TYPE "ST_SystemDataRef"
VERSION : 0.1


  STRUCT
   abyInputData : ARRAY  [1 .. 104 ] OF //This array contains the mapped raw input data
   BYTE ;
   abyOutputData : ARRAY  [1 .. 104 ] OF //This array contains the mapped raw output data
   BYTE ;
   stConnectionSettings : "ST_ConnectionSettings";	//This structure contains all data required for the connection
   xConnected : BOOL ;	//Connection established | FALSE: No connection established | TRUE: Connection es
   xStatusOfConnection : BOOL ;	//Status of the communication module | FALSE: No connection established | TRUE: C
   byActualComMode : BYTE ;	//Actual communication mode | 0x00 = Acyclic communication mode | 0x01 = Cyclic c
   byActualAccessType : BYTE ;	//Actual access type | 0x00 = Read object | 0x01 = Write object
   stAcyclicReadRequest : "ST_AcyclicReadRequest";	//This structure contains all data required to create a acyclic read request
   stAcyclicReadResponse : "ST_AcyclicReadResponse";	//This structure contains all data required to parse a acyclic read response
   stAcyclicWriteRequest : "ST_AcyclicWriteRequest";	//This structure contains all data required to create a acyclic write request
   stAcyclicWriteResponse : "ST_AcyclicWriteResponse";	//This structure contains all data required to parse a acyclic write response
   stCyclicRequest : "ST_CyclicRequest";	//This structure contains all data required to create a cyclic request
   stCyclicResponse : "ST_CyclicResponse";	//This structure contains all data required to parse a cyclic response
  END_STRUCT ;
END_TYPE

